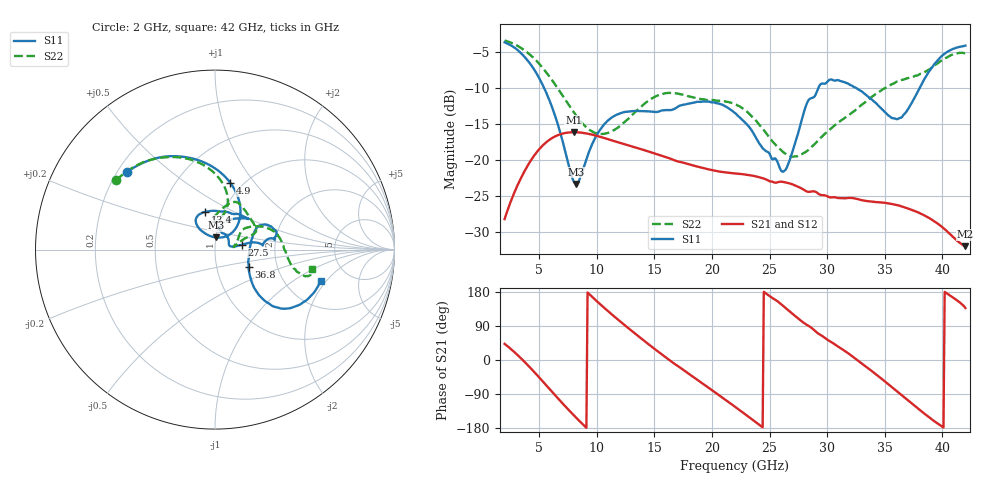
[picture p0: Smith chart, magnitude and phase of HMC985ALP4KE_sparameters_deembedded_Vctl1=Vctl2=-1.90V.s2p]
!s2p File: Measurements: S11, S21, S12, S22
# GHz S dB R 50.0
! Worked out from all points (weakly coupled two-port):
!   401 points, 2 GHz to 42 GHz, reference 50 ohm
!   highest |S21| = -16.19 dB at 8 GHz (marker M1); lowest = -32.0 dB at 42 GHz (marker M2)
!   lowest |S11| = -23.4 dB at 8.2 GHz (marker M3), VSWR 1.15, Z = 50.3 + j6.81 ohm
!   |S11| at or under -10 dB: 5.413 GHz to 29.25 GHz (23.84 GHz wide, 138 % of centre); 32.45 GHz to 38.04 GHz (5.595 GHz wide, 15.9 % of centre)
!   |S22| runs from -19.6 to -3.5 dB; largest |S21 - S12| = 0.00016
!   S11 on the Smith chart (normalised r, x): 2 GHz: 0.24, +0.36; 4.9 GHz: 0.88, +0.76; 13.4 GHz: 0.82, +0.36; 27.5 GHz: 1.36, +0.08; 36.8 GHz: 1.43, -0.29; 42 GHz: 3.13, -1.80
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2  -3.71 138.4  -28.26 42.6  -28.27 42.6  -3.45 144.9
3.4  -5.19 109.8  -22.64 5.1  -22.64 5.1  -4.47 121.4
4.9  -8.38 77.0  -18.75 -42.5  -18.75 -42.5  -6.51 97.3
6.1  -12.63 53.1  -17.03 -83.3  -17.03 -83.3  -8.92 81.8
8  -23.04 71.7  -16.19 -145.7  -16.20 -145.7  -13.41 75.1
8.2  -23.37 83.9  -16.20 -151.9  -16.20 -151.9  -13.86 76.1
8.7  -21.90 109.7  -16.27 -167.1  -16.27 -167.1  -14.87 79.8
10.7  -15.01 125.8  -17.02 136.2  -17.03 136.2  -16.41 96.5
13.4  -13.24 105.0  -18.34 67.9  -18.35 67.9  -13.29 83.4
15.4  -13.32 79.3  -19.35 20.5  -19.35 20.5  -11.02 69.7
18.9  -11.98 43.7  -21.04 -55.9  -21.04 -55.9  -11.54 44.2
22  -13.53 55.4  -21.91 -123.3  -21.92 -123.3  -12.30 22.7
24.5  -18.56 80.2  -22.64 179.9  -22.64 180.0  -15.91 18.9
26.1  -21.68 19.7  -23.08 144.7  -23.09 144.7  -18.84 10.7
27.5  -16.22 10.3  -23.79 109.1  -23.78 109.1  -19.45 8.3
28.7  -11.43 5.2  -24.41 83.4  -24.42 83.4  -18.16 17.3
31.1  -9.06 17.5  -25.35 32.6  -25.36 32.5  -14.69 35.4
33.3  -10.91 28.3  -25.72 -15.9  -25.73 -16.0  -12.04 30.9
35.4  -13.96 8.4  -26.10 -66.1  -26.11 -66.1  -9.73 20.4
36.8  -13.50 -27.5  -26.68 -101.1  -26.68 -101.0  -8.78 11.0
39.7  -6.00 -41.1  -29.02 -169.8  -29.03 -170.0  -6.51 -15.1
42  -4.17 -16.6  -32.02 137.1  -32.00 137.1  -5.19 -11.4
